(* Logix 5000 AddOnInstructionDefinition export EH_Nivector_FTI26_IOL; software revision 38.00 *)

TYPE EH_CommAOI_Data :
STRUCT
   Device_Comm_Error : BOOL;
   CommSuccess : BOOL;
   CommFailed : BOOL;
   CommTimeOut : BOOL;
   StateDone : BOOL;
   NewState : BOOL;
   OldState : SINT;
   PortSize : SINT;
   DevicePort : SINT;
   MaxState : SINT;
   State : SINT;
   VendorID : INT;
   DeviceID : DINT;
   CyclicData : INT[16];
   AcyclicData : DINT[8];
   ReplayIndex : INT;
   AOI_Diagnostic : DINT;
   ConnectionStatus : DINT;
   OutputData : INT[16];
END_STRUCT
END_TYPE

ADD_ON_INSTRUCTION EH_Nivector_FTI26_IOL   (* revision 1.0, vendor Endress+Hauser *)
// Nivector FTI26 Rev 1 IO-Link
// Nivector FTI26 Rev 2 IO-Link
VAR_IN_OUT
   DataToSend : INT[10]; {required}
   CommAOIBusy : DINT; {required}
   ActiveComPort : DINT; {required}
   DeviceAOISendRequest : DINT; {required}
   CommError : INT; {required}
   DeviceData : EH_CommAOI_Data; {required}
END_VAR
VAR_INPUT
   iExecuteRisingEdge : BOOL; {visible}
   iSetSimulation_Q1 : SINT; {visible}
   iSetSimulation_Q2 : SINT; {visible}
END_VAR
VAR_OUTPUT
   qVendor_ID : DINT; {access Read Only, visible}
   qDevice_ID : DINT; {access Read Only, visible}
   qCoverage : REAL; {visible}
   qS_Out_1 : BOOL; {access Read Only, visible}
   qSimulationActiveQ1 : SINT; {visible}
   qS_Out_2 : BOOL; {access Read Only, visible}
   qSimulationActiveQ2 : SINT; {access Read Only, visible}
   qAOI_Diagnostic : DINT; {access Read Only, visible}
END_VAR
VAR_IN_OUT
   qActual_Diagnostics_String : STRING; {required}
END_VAR
VAR_OUTPUT
   qActual_Diagnostics_Code : DINT; {access Read Only, visible}
END_VAR
VAR_IN_OUT
   qLast_Diagnostics_String : STRING; {required}
END_VAR
VAR_OUTPUT
   qLast_Diagnostics_Code : DINT; {access Read Only, visible}
   qCommunicationBusy : DINT; {visible}
   qCommError : DINT; {access None, visible}
   qDeviceConnectionError : BOOL; {access Read Only, visible}
END_VAR
VAR_INPUT
   DeviceID1 : DINT;
   DeviceID2 : DINT;
   qDevice_ID_select : INT;
END_VAR
VAR
   Calc_DID : DINT; {access None}
   Calc_VID : DINT; {access None}
   Coverage_DINT : DINT; {access None}
   Calc_Coverage : DINT; {access None}
   Calc_CondenStatus : DINT; {access None}
   CMD_Index : INT; {access None}
   CMD_Subindex : INT; {access None}
   CMD_ByteLength : INT; {access None}
   oldCondStatus : USINT; {access None}
   Trigger : BOOL; {access None}
   CMD_Rd : BOOL; {access None}
   CMD_Wr : BOOL; {access None}
   Calc_Out : DINT; {access None}
   UnitSelection : REAL; {access None}
   InputByteLength : DINT;
   StateMin : DINT; {access None}
   UseDeviceUnit : BOOL; {access None}
   ActiveAOI : BOOL; {access None}
   firstTimeDone : BOOL; {access None}
   AOI_Prio : BOOL; {access None}
   CondStatusChanged : BOOL; {access None}
   FALSE : BOOL; {access None}
   TRUE : BOOL := 1; {access None}
END_VAR

ROUTINE Logic   (* structured text *)
// PMP23 Communication via AL1323
   // =======================================================================
   // Endress+Hauser Digital Solutions
   // ©Copyright (2024) All Rights Reserved
   // =======================================================================
   // Name:                EH_Nivector_FTI26_IOL
   // Version:             1.0
   // Datum:               11.2025
   // Library:             01.01.00
   // Engineering:         Studio5000 V38.00.00
   // Author:              EH
   // =======================================================================
   
   
   qAOI_Diagnostic := DeviceData.AOI_Diagnostic;
   qCommunicationBusy := CommAOIBusy;
   DeviceID1 := 768;
   DeviceID2 := 769;
   StateMin := 0;
   DeviceData.MaxState := 7;
   
   if DeviceData.DevicePort = 0 or DeviceData.DeviceID < DeviceID1 or DeviceData.DeviceID > DeviceID2 or DeviceData.ConnectionStatus <> 1 then
   
   	qVendor_ID	:= 0;
   	qDevice_ID	:= 0;
   	qCoverage	:= 0;
   	qS_Out_1	:= 0;
   	qS_Out_2	:= 0;
   	qSimulationActiveQ1	:= 0;
   	qActual_Diagnostics_Code	:= 0;
   	qLast_Diagnostics_Code	:= 0;
   	qLast_Diagnostics_String	:= '';
   
   	if DeviceData.DevicePort = 0 then
   
   		qActual_Diagnostics_String	:= 'Device Port is Zero';
   		DeviceData.AOI_Diagnostic.1 := TRUE;
   
   	elsif DeviceData.ConnectionStatus <> 1 then
   
   		qActual_Diagnostics_String	:= 'No Device connected';
   		qDeviceConnectionError := TRUE;
   
   	elsif DeviceData.DeviceID < DeviceID1 or DeviceData.DeviceID > DeviceID2  then
   
   		qActual_Diagnostics_String	:= 'Wrong DeviceID';
   		DeviceData.AOI_Diagnostic.2 := TRUE;
   		qVendor_ID := DeviceData.VendorID;
   		qDevice_ID := DeviceData.DeviceID;
   
   	end_if;
   
   else
   
   	if qActual_Diagnostics_Code = 0 then
   
   		qActual_Diagnostics_String	:= '--------';
   
   	end_if;
   
   	if qLast_Diagnostics_Code = 0 then
   
   		qLast_Diagnostics_String	:= '--------';
   
   	end_if;
   
   	DeviceData.AOI_Diagnostic.1 := FALSE;
   	qDeviceConnectionError := FALSE;
   	DeviceData.AOI_Diagnostic.2  := FALSE;
   
   end_if;
   
   
   if not DeviceData.AOI_Diagnostic.0
   	and not qDeviceConnectionError
   	and not DeviceData.AOI_Diagnostic.2
   	and DeviceData.DevicePort > 0 or ActiveAOI and qDeviceConnectionError then
   
   	//*********************************
   	//Vendor ID
   	//*********************************
   
   	qVendor_ID := DeviceData.VendorID;
   
   	//*********************************
   	//Device ID
   	//*********************************
   
   	qDevice_ID := DeviceData.DeviceID;
   
   	if DeviceData.DeviceID = DeviceID1 then
   
   		qDevice_ID_select :=1;
   
   	elsif DeviceData.DeviceID = DeviceID2 then
   
   		qDevice_ID_select := 2;
   
   	else
   
   		qDevice_ID_select := 0;
   
   	end_if;
   
   	Calc_Coverage := 0+((DeviceData.DevicePort-1)*InputByteLength);
   
   	case qDevice_ID_select of  // check for Different Version
   
   		//*********************************
   	    1: // Nivector Rev.1
   	    //*********************************
   
   		Coverage_DINT.0 := DeviceData.CyclicData[Calc_Coverage].0;
   		Coverage_DINT.1 := DeviceData.CyclicData[Calc_Coverage].1;
   		Coverage_DINT.2 := DeviceData.CyclicData[Calc_Coverage].2;
   		Coverage_DINT.3 := DeviceData.CyclicData[Calc_Coverage].3;
   		Coverage_DINT.4 := DeviceData.CyclicData[Calc_Coverage].4;
   		Coverage_DINT.5 := DeviceData.CyclicData[Calc_Coverage].5;
   		Coverage_DINT.6 := DeviceData.CyclicData[Calc_Coverage].6;
   		Coverage_DINT.7	:= DeviceData.CyclicData[Calc_Coverage].7;
   		Coverage_DINT.8 := DeviceData.CyclicData[Calc_Coverage].8;
   		Coverage_DINT.9 := DeviceData.CyclicData[Calc_Coverage].9;
   		Coverage_DINT.10 := DeviceData.CyclicData[Calc_Coverage].10;
   		Coverage_DINT.11 := DeviceData.CyclicData[Calc_Coverage].11;
   		Coverage_DINT.12 := DeviceData.CyclicData[Calc_Coverage].12;
   		Coverage_DINT.13 := DeviceData.CyclicData[Calc_Coverage].13;
   		Coverage_DINT.14 := DeviceData.CyclicData[Calc_Coverage].13;
   		Coverage_DINT.15 := DeviceData.CyclicData[Calc_Coverage].13;
   		Coverage_DINT.16 := DeviceData.CyclicData[Calc_Coverage].13;
   		Coverage_DINT.17 := DeviceData.CyclicData[Calc_Coverage].13;
   		Coverage_DINT.18 := DeviceData.CyclicData[Calc_Coverage].13;
   		Coverage_DINT.19 := DeviceData.CyclicData[Calc_Coverage].13;
   		Coverage_DINT.20 := DeviceData.CyclicData[Calc_Coverage].13;
   		Coverage_DINT.21 := DeviceData.CyclicData[Calc_Coverage].13;
   		Coverage_DINT.22 := DeviceData.CyclicData[Calc_Coverage].13;
   		Coverage_DINT.23 := DeviceData.CyclicData[Calc_Coverage].13;
   		Coverage_DINT.24 := DeviceData.CyclicData[Calc_Coverage].13;
   		Coverage_DINT.25 := DeviceData.CyclicData[Calc_Coverage].13;
   		Coverage_DINT.26 := DeviceData.CyclicData[Calc_Coverage].13;
   		Coverage_DINT.27 := DeviceData.CyclicData[Calc_Coverage].13;
   		Coverage_DINT.28 := DeviceData.CyclicData[Calc_Coverage].13;
   		Coverage_DINT.29 := DeviceData.CyclicData[Calc_Coverage].13;
   		Coverage_DINT.30 := DeviceData.CyclicData[Calc_Coverage].13;
   		Coverage_DINT.31 := DeviceData.CyclicData[Calc_Coverage].13;
   
   		qCoverage := Coverage_DINT;
   
   
   		//*********************************
   	    2: // Nivector Rev.2
   	    //*********************************
   
   		Coverage_DINT.0 := DeviceData.CyclicData[Calc_Coverage].0;
   		Coverage_DINT.1 := DeviceData.CyclicData[Calc_Coverage].1;
   		Coverage_DINT.2 := DeviceData.CyclicData[Calc_Coverage].2;
   		Coverage_DINT.3 := DeviceData.CyclicData[Calc_Coverage].3;
   		Coverage_DINT.4 := DeviceData.CyclicData[Calc_Coverage].4;
   		Coverage_DINT.5 := DeviceData.CyclicData[Calc_Coverage].5;
   		Coverage_DINT.6 := DeviceData.CyclicData[Calc_Coverage].6;
   		Coverage_DINT.7	:= DeviceData.CyclicData[Calc_Coverage].7;
   		Coverage_DINT.8 := DeviceData.CyclicData[Calc_Coverage].8;
   		Coverage_DINT.9 := DeviceData.CyclicData[Calc_Coverage].9;
   		Coverage_DINT.10 := DeviceData.CyclicData[Calc_Coverage].10;
   		Coverage_DINT.11 := DeviceData.CyclicData[Calc_Coverage].11;
   		Coverage_DINT.12 := DeviceData.CyclicData[Calc_Coverage].12;
   		Coverage_DINT.13 := DeviceData.CyclicData[Calc_Coverage].13;
   		Coverage_DINT.14 := DeviceData.CyclicData[Calc_Coverage].13;
   		Coverage_DINT.15 := DeviceData.CyclicData[Calc_Coverage].13;
   		Coverage_DINT.16 := DeviceData.CyclicData[Calc_Coverage].13;
   		Coverage_DINT.17 := DeviceData.CyclicData[Calc_Coverage].13;
   		Coverage_DINT.18 := DeviceData.CyclicData[Calc_Coverage].13;
   		Coverage_DINT.19 := DeviceData.CyclicData[Calc_Coverage].13;
   		Coverage_DINT.20 := DeviceData.CyclicData[Calc_Coverage].13;
   		Coverage_DINT.21 := DeviceData.CyclicData[Calc_Coverage].13;
   		Coverage_DINT.22 := DeviceData.CyclicData[Calc_Coverage].13;
   		Coverage_DINT.23 := DeviceData.CyclicData[Calc_Coverage].13;
   		Coverage_DINT.24 := DeviceData.CyclicData[Calc_Coverage].13;
   		Coverage_DINT.25 := DeviceData.CyclicData[Calc_Coverage].13;
   		Coverage_DINT.26 := DeviceData.CyclicData[Calc_Coverage].13;
   		Coverage_DINT.27 := DeviceData.CyclicData[Calc_Coverage].13;
   		Coverage_DINT.28 := DeviceData.CyclicData[Calc_Coverage].13;
   		Coverage_DINT.29 := DeviceData.CyclicData[Calc_Coverage].13;
   		Coverage_DINT.30 := DeviceData.CyclicData[Calc_Coverage].13;
   		Coverage_DINT.31 := DeviceData.CyclicData[Calc_Coverage].13;
   
   		qCoverage := Coverage_DINT;
   
   	end_case;
   
   	//*********************************
   	// Process Parameter State IO1
   	//*********************************
   
   		qS_Out_1 := DeviceData.CyclicData[Calc_Coverage].14;
   		qS_Out_2 := DeviceData.CyclicData[Calc_Coverage].15;
   
   
   	//*********************************
   	// Checking for CommBlockBusy
   	//*********************************
   
   	if iExecuteRisingEdge and DeviceData.State = 0 and not ActiveAOI then
   		DeviceAOISendRequest.[DeviceData.DevicePort] := 1;
   
   	end_if;
   
   
   	if ActiveComPort = DeviceData.DevicePort then
   
   		AOI_Prio :=1;
   	else
   
   		AOI_Prio := 0;
   	end_if;
   
   
   	if CommAOIBusy = 1 and iExecuteRisingEdge and DeviceData.State = 0 and AOI_Prio and not ActiveAOI then
   
   		ActiveAOI := 1;
   
   	end_if;
   
   	qCommunicationBusy := CommAOIBusy;
   	qAOI_Diagnostic :=DeviceData.AOI_Diagnostic;
   
   	if  ActiveAOI and qDeviceConnectionError then
   
   		DeviceData.State := DeviceData.MaxState;
   
   	end_if;
   
   	//*********************************
   	// State machine
   	//*********************************
   
   
   	if ActiveAOI or DeviceData.State = DeviceData.MaxState then
   
   	case DeviceData.State of
   
   	    //*********************************
   	    0: // Idle
   	    //*********************************
   
   	    // Initializing
   	   		Trigger := 0;
   		    CMD_Index := 0;
   			CMD_Subindex := 0;
   	        CMD_Wr := 0;
   			CMD_Rd := 0;
   	        CMD_ByteLength := 0;
   
   			if DeviceData.DevicePort = ActiveComPort then
   					DeviceData.CommSuccess := 0;
   					DeviceData.CommTimeOut := 0;
   					DeviceData.NewState := 1;
   					DeviceData.StateDone := 0;
   			end_if;
   
   			// Wait for trigger
   			if iExecuteRisingEdge and ActiveComPort = DeviceData.DevicePort then
   
   				DeviceData.AOI_Diagnostic := 0;
   				DeviceData.State := DeviceData.State + 1;
   
   			end_if;
   
   
   		//*********************************
   		1: // Set Simulation Q1
   		//*********************************
   
   	        CMD_Index := 89;
   	        CMD_Subindex := 0;
   	        CMD_Wr := 1;
   			CMD_Rd := 0;
   	        CMD_ByteLength := 1;
   			DataToSend[6]:= 0;
   			DataToSend[7]:= 0;
   			qAOI_Diagnostic.8 := 0;
   
   			if iSetSimulation_Q1 >=0 and iSetSimulation_Q1 <=2 then
   
   				DataToSend[6] := iSetSimulation_Q1;
   				Trigger := 1;
   
   				if DeviceData.NewState then
   
   					DeviceData.StateDone := 1;
   
   				end_if;
   
   
   				if  DeviceData.CommSuccess and DeviceData.ReplayIndex = CMD_Index then
   
   					Trigger := 0;
   					DeviceData.OldState := DeviceData.State;
   					DeviceData.State := DeviceData.State + 1;
   					DeviceData.CommSuccess := 0;
   					DeviceData.AcyclicData[0] := 0;
   					DeviceData.NewState := 1;
   
   			 	elsif DeviceData.CommTimeOut then
   
   					DeviceData.AOI_Diagnostic.[DeviceData.State+7] := 1;
   					DeviceData.OldState := DeviceData.State;
   		        	DeviceData.State := DeviceData.State + 1;
   					DeviceData.CommTimeOut := 0;
   					DeviceData.AcyclicData[0] := 0;
   					DeviceData.NewState := 1;
   
   		    	end_if;
   
   			else
   
   				DeviceData.AOI_Diagnostic.[DeviceData.State+7] := 1;
   				DeviceData.OldState := DeviceData.State;
   		        DeviceData.State := DeviceData.State + 1;
   				DeviceData.CommTimeOut := 0;
   				DeviceData.AcyclicData[0] := 0;
   				DeviceData.NewState := 1;
   
   			end_if;
   
   	    //*********************************
   	    2: // Set Simulation Q2
   	    //*********************************
   
   	        CMD_Index := 68;
   	        CMD_Subindex := 0;
   	        CMD_Wr := 1;
   			CMD_Rd := 0;
   	        CMD_ByteLength := 1;
   			DataToSend[6]:= 0;
   			DataToSend[7]:= 0;
   
   			if iSetSimulation_Q2 >=0 and iSetSimulation_Q2 <=2 then
   
   				DataToSend[6] := iSetSimulation_Q2;
   				Trigger := 1;
   
   				if DeviceData.NewState then
   					DeviceData.StateDone := 1;
   				end_if;
   
   				if  DeviceData.CommSuccess and DeviceData.ReplayIndex = CMD_Index then
   
   					Trigger := 0;
   					DeviceData.OldState := DeviceData.State;
   					DeviceData.State := DeviceData.State + 1;
   					DeviceData.CommSuccess := 0;
   					DeviceData.AcyclicData[0] := 0;
   					DeviceData.NewState := 1;
   
   			 	elsif DeviceData.CommTimeOut then
   
   					DeviceData.AOI_Diagnostic.[DeviceData.State+7] := 1;
   					DeviceData.OldState := DeviceData.State;
   		        	DeviceData.State := DeviceData.State + 1;
   					DeviceData.CommTimeOut := 0;
   					DeviceData.AcyclicData[0] := 0;
   					DeviceData.NewState := 1;
   
   		    	end_if;
   
   			else
   
   				DeviceData.AOI_Diagnostic.[DeviceData.State+7] := 1;
   				DeviceData.OldState := DeviceData.State;
   		        DeviceData.State := DeviceData.State + 1;
   				DeviceData.CommTimeOut := 0;
   				DeviceData.AcyclicData[0] := 0;
   				DeviceData.NewState := 1;
   
   			end_if;
   
   		//*********************************
   	    3: // Read Simulation Active Q1
   	    //*********************************
   
   			CMD_Index := 89;
   	        CMD_Subindex := 0;
   	        CMD_Wr := 0;
   			CMD_Rd := 1;
   	        CMD_ByteLength := 1;
   			DataToSend[6]:= 0;
   			DataToSend[7]:= 0;
   			Trigger := 1;
   
   			if DeviceData.NewState then
   
   				DeviceData.StateDone := 1;
   
   			end_if;
   
   			if  DeviceData.CommSuccess and DeviceData.ReplayIndex = CMD_Index then
   
   
   				qSimulationActiveQ1 := DeviceData.AcyclicData[0];
   
   					Trigger := 0;
   					DeviceData.OldState := DeviceData.State;
   					DeviceData.State := DeviceData.State + 1;
   					DeviceData.CommSuccess := 0;
   					DeviceData.AcyclicData[0] := 0;
   					DeviceData.NewState := 1;
   
   			 elsif DeviceData.CommTimeOut then
   
   					DeviceData.AOI_Diagnostic.[DeviceData.State+7] := 1;
   					DeviceData.OldState := DeviceData.State;
   		        	DeviceData.State := DeviceData.State + 1;
   					DeviceData.CommTimeOut := 0;
   					DeviceData.AcyclicData[0] := 0;
   					DeviceData.NewState := 1;
   
   			end_if;
   
   		//*********************************
   	    4: // Read Simulation Active Q2
   	    //*********************************
   
   			CMD_Index := 68;
   	        CMD_Subindex := 0;
   	        CMD_Wr := 0;
   			CMD_Rd := 1;
   	        CMD_ByteLength := 1;
   			DataToSend[6]:= 0;
   			DataToSend[7]:= 0;
   			Trigger := 1;
   
   			if DeviceData.NewState then
   
   				DeviceData.StateDone := 1;
   
   			end_if;
   
   			if  DeviceData.CommSuccess and DeviceData.ReplayIndex = CMD_Index then
   
   				qSimulationActiveQ2 := DeviceData.AcyclicData[0];
   
   				Trigger := 0;
   				DeviceData.OldState := DeviceData.State;
   				DeviceData.State := DeviceData.State + 1;
   				DeviceData.CommSuccess := 0;
   				DeviceData.AcyclicData[0] := 0;
   				DeviceData.NewState := 1;
   
   			elsif DeviceData.CommTimeOut then
   
   				DeviceData.AOI_Diagnostic.[DeviceData.State+7] := 1;
   				DeviceData.OldState := DeviceData.State;
   		       	DeviceData.State := DeviceData.State + 1;
   				DeviceData.CommTimeOut := 0;
   				DeviceData.AcyclicData[0] := 0;
   				DeviceData.NewState := 1;
   
   		   	end_if;
   
   		//*********************************
   	    5: // Actual Diagnostic
   	    //*********************************
   
   	        CMD_Index := 260;
   	        CMD_Subindex := 0;
   	        CMD_Wr := 0;
   			CMD_Rd := 1;
   			CMD_ByteLength := 2;
   
   			Trigger := 1;
   
   			if DeviceData.NewState then
   
   				DeviceData.StateDone := 1;
   
   			end_if;
   
   			if  DeviceData.CommSuccess and DeviceData.ReplayIndex = CMD_Index then
   
   				qActual_Diagnostics_Code	:= DeviceData.AcyclicData[0];
   
   				case qActual_Diagnostics_Code of
   
   		        16#2D2D_2D2D:
   		           qActual_Diagnostics_String := 'SYSTEM OK';
   				16#0000_0001:
   					qActual_Diagnostics_String := 'no communication';
   				16#4632_3730:
   				    qActual_Diagnostics_String := 'F270 - Defect in electronic / sensor';
   				16#5338_3034:
   				    qActual_Diagnostics_String := 'S804 - Load current > 200mA per output';
   				16#4D32_3930:
   				    qActual_Diagnostics_String := 'M290 - Device wiring fault';
   				16#4334_3835:
   				    qActual_Diagnostics_String := 'C485 - Simulation active';
   				16#4331_3832:
   				    qActual_Diagnostics_String := 'C182 - Invalid calibration';
   				16#4331_3033:
   				    qActual_Diagnostics_String := 'C103 - Sensor check failed';
   				16#5338_3235:
   				    qActual_Diagnostics_String := 'S825 - Ambient temperature out of specification';
   				else
   					qActual_Diagnostics_String := 'Error Code unknown';
   
   		 		end_case;
   
   				Trigger := 0;
   				DeviceData.OldState := DeviceData.State;
   		        DeviceData.State := DeviceData.State + 1;
   				DeviceData.CommSuccess := 0;
   				DeviceData.AcyclicData[0] := 0;
   				DeviceData.NewState := 1;
   
   
   
   			 elsif DeviceData.CommTimeOut then
   
   				DeviceData.AOI_Diagnostic.[DeviceData.State+7] := 1;
   				DeviceData.OldState := DeviceData.State;
   		        DeviceData.State := DeviceData.State + 1;
   				DeviceData.CommTimeOut := 0;
   				DeviceData.AcyclicData[0] := 0;
   				DeviceData.NewState := 1;
   
   		    end_if;
   
   		//*********************************
   	    6: // Last Diagnostic
   	    //*********************************
   
   	        CMD_Index := 261;
   			CMD_Subindex := 0;
   	        CMD_Wr := 0;
   			CMD_Rd := 1;
   			CMD_ByteLength := 2;
   	        Trigger := 1;
   			if DeviceData.NewState then
   				DeviceData.StateDone := 1;
   			end_if;
   
   			if  DeviceData.CommSuccess and DeviceData.ReplayIndex = CMD_Index then
   
   				qLast_Diagnostics_Code	:= DeviceData.AcyclicData[0];
   
   				case qLast_Diagnostics_Code of
   
   		        16#2D2D_2D2D:
   		           qLast_Diagnostics_String := 'SYSTEM OK';
   				16#0000_0001:
   					qLast_Diagnostics_String := 'no communication';
   				16#4632_3730:
   				    qLast_Diagnostics_String := 'F270 - Defect in electronic / sensor';
   				16#5338_3034:
   				    qLast_Diagnostics_String := 'S804 - Load current > 200mA per output';
   				16#4D32_3930:
   				    qLast_Diagnostics_String := 'M290 - Device wiring fault';
   				16#4334_3835:
   				    qLast_Diagnostics_String := 'C485 - Simulation active';
   				16#4331_3832:
   				    qLast_Diagnostics_String := 'C182 - Invalid calibration';
   				16#4331_3033:
   				    qLast_Diagnostics_String := 'C103 - Sensor check failed';
   				16#5338_3235:
   				    qLast_Diagnostics_String := 'S825 - Ambient temperature out of specification';
   				else
   					qLast_Diagnostics_String := 'Error Code unknown';
   
   		 		end_case;
   
   				Trigger := 0;
   				DeviceData.OldState := DeviceData.State;
   		        DeviceData.State := DeviceData.State + 1;
   				DeviceData.CommSuccess := 0;
   				DeviceData.AcyclicData[0] := 0;
   				DeviceData.NewState := 1;
   
   
   
   			 elsif DeviceData.CommTimeOut then
   
   				DeviceData.AOI_Diagnostic.[DeviceData.State+7] := 1;
   				DeviceData.OldState := DeviceData.State;
   		        DeviceData.State := DeviceData.State + 1;
   				DeviceData.CommTimeOut := 0;
   				DeviceData.AcyclicData[0] := 0;
   				DeviceData.NewState := 1;
   
   		    end_if;
   
   		//*********************************
   	    7: // Trigger guard
   	    //*********************************
   
   			if not firstTimeDone then
   
   				CommAOIBusy := 0;
   				firstTimeDone := 1;
   				DeviceAOISendRequest.[DeviceData.DevicePort] := 0;
   				ActiveComPort := 0;
   				ActiveAOI := 0;
   				DataToSend[0] := 0;
   				DataToSend[1] := 0;
   				DataToSend[2] := 0;
   				DataToSend[3] := 0;
   				DataToSend[4] := 0;
   				DataToSend[5] := 0;
    				DataToSend[6] := 0;
   				DataToSend[7] := 0;
   				DataToSend[8] := 0;
   				DataToSend[9] := 0;
   				DeviceData.StateDone := 0;
   
   
   			end_if;
   
   			if DeviceData.State =  DeviceData.MaxState AND NOT iExecuteRisingEdge then
   
   				DeviceData.State := 0;
   				DeviceData.OldState := DeviceData.State;
   				firstTimeDone := 0;
   
   			end_if;
   
   	end_case;
   
   	end_if;
   
   
   	//*************************
   	// Write Commands to the Master and the Device
   	//*************************
   	if DeviceData.State > StateMin and DeviceData.State < DeviceData.MaxState then
   
   	DataToSend[2] := DeviceData.DevicePort;
   	DataToSend[3] := CMD_Index;
   	DataToSend[4] := CMD_Subindex;
   	DataToSend[5].0 := CMD_Rd;
   	DataToSend[5].1 := CMD_Wr;
   	DataToSend[5].8 := CMD_ByteLength.0;
   	DataToSend[5].9 := CMD_ByteLength.1;
   	DataToSend[5].10 := CMD_ByteLength.2;
   	DataToSend[5].11 := CMD_ByteLength.3;
   	DataToSend[5].12 := CMD_ByteLength.4;
   	DataToSend[5].13 := CMD_ByteLength.5;
   	DataToSend[5].14 := CMD_ByteLength.6;
   	DataToSend[5].15 := CMD_ByteLength.7;
   
   	DataToSend[5].7 := Trigger;
   
   	qCommError := CommError;
   
   	end_if;
   
   end_if;
END_ROUTINE
END_ADD_ON_INSTRUCTION
